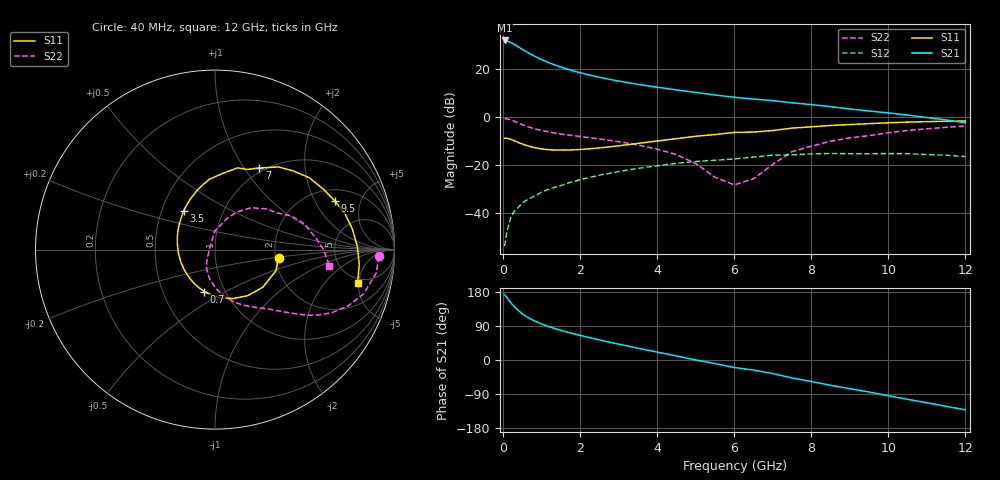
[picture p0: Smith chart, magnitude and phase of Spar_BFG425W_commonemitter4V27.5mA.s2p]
! Filename: 427bfg415.001
! BFG425W Field C1
! V1=8.367E-001V,V2=4.000E+000V, I1=3.438E-004A, I2=2.747E-002A
# GHz  S  MA  R 50
!  S11  S21  S12  S22
!Freq(GHz)  Mag  Ang  Mag  Ang  Mag  Ang  Mag  Ang
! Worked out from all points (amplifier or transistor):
!   44 points, 40 MHz to 12 GHz, reference 50 ohm
!   highest |S21| = 31.9 dB at 40 MHz (marker M1)
!   |S21| within 3 dB of that: start of sweep to 431.3 MHz
!   unconditionally stable (mu >= 1): start of sweep to 47.8 MHz; 1.191 GHz to end of sweep
!   at 700 MHz: K = 0.83, MSG = 30.1 dB, |S12| = -34.0 dB
!   at 2.4 GHz: K = 1.15, MAG = 18.4 dB, |S12| = -24.7 dB
!   at 12 GHz: K = 1.34, MAG = 3.6 dB, |S12| = -16.6 dB
!   S11 on the Smith chart (normalised r, x): 40 MHz: 2.08, -0.21; 700 MHz: 0.80, -0.40; 3.5 GHz: 0.65, +0.31; 7 GHz: 0.95, +1.18; 9.5 GHz: 2.59, +2.94; 12 GHz: 4.39, -4.85
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0.04  0.357 -7.2  39.21 172.8  0.002 60.5  0.913 -2.4
0.1  0.359 -19.4  38.19 164.7  0.004 75.3  0.908 -8.2
0.2  0.339 -38.2  35.59 151.2  0.008 72.9  0.864 -16.6
0.3  0.315 -54.5  32.15 140.0  0.011 70.3  0.803 -23.2
0.4  0.291 -69.6  28.77 130.3  0.013 67.4  0.742 -28.1
0.5  0.271 -83.0  25.68 121.8  0.016 65.5  0.688 -31.9
0.6  0.254 -94.3  22.97 115.0  0.018 64.6  0.641 -34.8
0.7  0.241 -104.4  20.68 109.2  0.02 63.5  0.602 -37.0
0.9  0.221 -122.1  17.08 99.3  0.024 62.3  0.542 -40.5
1.2  0.206 -143.0  13.39 87.8  0.031 60.4  0.482 -44.8
1.6  0.202 -165.3  10.3 75.5  0.039 57.7  0.428 -49.9
2.2  0.214 169.1  7.595 60.1  0.053 51.9  0.371 -58.6
2.8  0.238 148.5  5.979 46.3  0.067 45.0  0.32 -68.0
3.5  0.279 128.7  4.765 31.3  0.084 35.7  0.259 -80.1
4.5  0.35 105.5  3.647 10.7  0.107 20.9  0.163 -101.3
5.5  0.427 84.2  2.859 -9.4  0.124 5.2  0.055 -137.6
6.5  0.481 68.2  2.351 -26.6  0.145 -7.0  0.051 110.1
7  0.518 61.4  2.177 -35.8  0.158 -14.6  0.102 91.2
8.5  0.66 37.5  1.631 -66.7  0.172 -44.0  0.309 49.1
9.5  0.72 22.3  1.322 -84.4  0.17 -60.7  0.405 30.1
10.5  0.774 8.5  1.089 -103.8  0.17 -79.3  0.518 16.0
12  0.816 -13.1  0.75 -131.3  0.148 -109.3  0.644 -8.1
